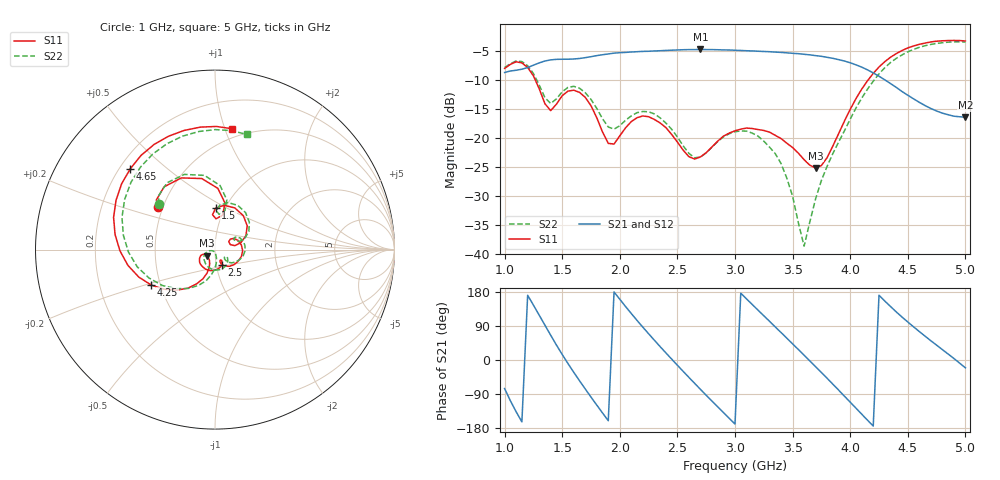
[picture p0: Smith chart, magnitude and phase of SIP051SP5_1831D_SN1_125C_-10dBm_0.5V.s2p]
# GHz  S  dB  R  50
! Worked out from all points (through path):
!   81 points, 1 GHz to 5 GHz, reference 50 ohm
!   highest |S21| = -4.81 dB at 2.7 GHz (marker M1); lowest = -16.4 dB at 5 GHz (marker M2)
!   lowest |S11| = -25.2 dB at 3.7 GHz (marker M3), VSWR 1.12, Z = 45.8 - j3.15 ohm
!   |S11| at or under -10 dB: 1.265 GHz to 4.157 GHz (2.892 GHz wide, 107 % of centre)
!   |S22| runs from -38.6 to -3.5 dB; largest |S21 - S12| = 0.0021
!   S11 on the Smith chart (normalised r, x): 1 GHz: 0.47, +0.26; 1.5 GHz: 0.90, +0.44; 2.5 GHz: 1.07, -0.18; 4.25 GHz: 0.44, -0.21; 4.65 GHz: 0.24, +0.38; 5 GHz: 0.42, +1.06
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1  -8.05 143.4  -8.76 -75.3  -8.77 -75.4  -7.90 140.7
1.2  -7.90 100.6  -7.92 170.8  -7.91 170.9  -7.58 98.1
1.35  -14.13 77.5  -6.79 92.0  -6.77 91.8  -13.09 75.7
1.5  -12.75 89.2  -6.49 14.5  -6.47 14.6  -12.08 83.9
1.7  -13.03 36.4  -6.21 -76.4  -6.22 -76.4  -12.23 38.6
1.8  -16.53 15.0  -5.86 -118.9  -5.86 -119.0  -14.92 21.2
1.95  -21.05 30.2  -5.44 179.7  -5.44 179.8  -18.49 28.5
2.15  -16.53 9.8  -5.19 104.3  -5.19 104.3  -15.66 16.1
2.35  -17.43 -39.0  -5.02 35.3  -5.00 35.5  -16.55 -21.8
2.5  -20.71 -65.0  -4.89 -13.9  -4.88 -13.9  -19.84 -43.8
2.7  -23.27 -58.8  -4.81 -77.5  -4.80 -77.4  -23.30 -33.4
2.85  -20.55 -68.5  -4.85 -123.6  -4.85 -123.6  -20.63 -39.7
3  -18.78 -90.9  -4.94 -168.9  -4.93 -169.0  -18.93 -66.9
3.15  -18.38 -116.6  -5.05 146.4  -5.05 146.4  -19.18 -100.4
3.35  -19.56 -145.4  -5.26 87.2  -5.26 87.2  -22.71 -147.9
3.6  -23.75 -156.7  -5.63 12.5  -5.63 12.6  -38.59 -121.6
3.7  -25.16 -141.6  -5.86 -17.7  -5.84 -17.7  -30.43 -80.6
3.95  -17.11 -108.8  -6.79 -95.5  -6.78 -95.3  -18.78 -92.8
4.25  -7.82 -150.9  -9.40 170.7  -9.38 170.5  -8.99 -145.7
4.35  -6.14 -169.8  -10.66 141.2  -10.66 141.0  -7.05 -167.6
4.65  -3.71 136.2  -14.44 62.9  -14.46 62.8  -4.16 132.1
5  -3.35 82.1  -16.44 -20.7  -16.44 -20.7  -3.54 74.6
